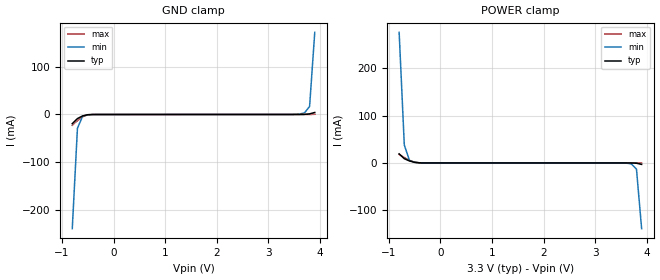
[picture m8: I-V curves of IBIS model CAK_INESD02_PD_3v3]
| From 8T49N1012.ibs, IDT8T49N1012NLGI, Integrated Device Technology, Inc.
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| 3.25758e+00   -2.17677e-02   -5.28452e-01   -1.11757e-02
| 3.33333e+00   -5.02723e-02   -7.41922e-01   -2.21158e-02
| 3.40909e+00   -2.62314e-01   -9.55756e-01   -3.46040e-02
| 3.48485e+00   -5.48303e-01   -1.16986e+00   -4.62037e-02
| 3.56061e+00   -8.34641e-01   -1.38418e+00   -9.03765e-02
| 3.63636e+00   -1.12130e+00   -1.59869e+00   -4.17028e-01
| 3.71212e+00   -1.40825e+00   -1.81339e+00   -7.83888e-01
| 3.78788e+00   -1.69546e+00   -2.02826e+00   -1.15108e+00
| 3.86364e+00   -1.98293e+00   -2.24329e+00   -1.51857e+00
| 3.93939e+00   -2.27062e+00   -2.45848e+00   -1.88632e+00
| 4.01515e+00   -2.55852e+00   -2.67383e+00   -2.25428e+00
| 4.09091e+00   -2.84661e+00   -2.88932e+00   -2.62244e+00
| 4.16667e+00   -3.13486e+00   -3.10494e+00   -2.99075e+00
| 4.24242e+00   -3.42327e+00   -3.32071e+00   -3.35921e+00
| 4.31818e+00   -3.71181e+00   -3.53659e+00   -3.72777e+00
| 4.39394e+00   -4.00047e+00   -3.75260e+00   -4.09645e+00
| 4.46970e+00   -4.28924e+00   -3.96871e+00   -4.46521e+00
| 4.54545e+00   -4.57811e+00   -4.18494e+00   -4.83406e+00
| 4.62121e+00   -4.86706e+00   -4.40126e+00   -5.20297e+00
| 4.69697e+00   -5.15608e+00   -4.61767e+00   -5.57195e+00
| 4.77273e+00   -5.44517e+00   -4.83417e+00   -5.94098e+00
| 4.84848e+00   -5.73432e+00   -5.05076e+00   -6.31005e+00
| 4.92424e+00   -6.02353e+00   -5.26742e+00   -6.67914e+00
| 5.00000e+00   -6.31277e+00   -5.48416e+00   -7.04826e+00
[Model] CAK_INESD02_PD_3v3
Model_type   Input
Polarity   Non-Inverting
Vinl = 0.8V
Vinh = 2.0V
|   typ   min   max
C_comp   2pF   1.5pF   2.5pF
|   typ   min   max
[Voltage range]   3.3V   3.135V   3.465V
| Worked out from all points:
|   GND clamp passes 1 mA (typ) near -0.52 V on its own axis
|   POWER clamp passes 1 mA (typ) near -0.47 V on its own axis
[GND_clamp]
|Voltage   I (typ)   I (min)   I (max)
|Note, modeling breaks down at 250mA and above.  This is well beyond the functional   |
|operating range of the device.  Should this scenario occur, catastrophic failure and   |
|possible damage to the device and/or board is of higher concern than the I-V curve   |
|behavior.  The IBIS checker will flag currents in excess of 10A with warnings.  Lines   |
|with currents in excess of 0.35 A have been commented out.  The points still remain|
|available to the user if the user desires to use them.   |
|-3.30000e+00   -9.17988e+00   -7.26773e+00   -1.13298e+01
|-3.20000e+00   -8.80345e+00   -6.98545e+00   -1.08492e+01
|-3.10000e+00   -8.42702e+00   -6.70323e+00   -1.03687e+01
|-3.00000e+00   -8.05061e+00   -6.42105e+00   -9.88820e+00
|-2.90000e+00   -7.67421e+00   -6.13893e+00   -9.40766e+00
|-2.80000e+00   -7.29783e+00   -5.85686e+00   -8.92712e+00
|-2.70000e+00   -6.92147e+00   -5.57486e+00   -8.44657e+00
|-2.60000e+00   -6.54514e+00   -5.29293e+00   -7.96602e+00
|-2.50000e+00   -6.16885e+00   -5.01107e+00   -7.48547e+00
|-2.40000e+00   -5.79260e+00   -4.72930e+00   -7.00493e+00
|-2.30000e+00   -5.41640e+00   -4.44761e+00   -6.52441e+00
|-2.20000e+00   -5.04025e+00   -4.16601e+00   -6.04391e+00
|-2.10000e+00   -4.66418e+00   -3.88451e+00   -5.56345e+00
|-2.00000e+00   -4.28819e+00   -3.60313e+00   -5.08304e+00
|-1.90000e+00   -3.91230e+00   -3.32186e+00   -4.60270e+00
|-1.80000e+00   -3.53652e+00   -3.04073e+00   -4.12245e+00
|-1.70000e+00   -3.16087e+00   -2.75973e+00   -3.64230e+00
|-1.60000e+00   -2.78537e+00   -2.47887e+00   -3.16225e+00
|-1.50000e+00   -2.41006e+00   -2.19818e+00   -2.68233e+00
|-1.40000e+00   -2.03494e+00   -1.91765e+00   -2.20257e+00
|-1.30000e+00   -1.66006e+00   -1.63729e+00   -1.72300e+00
|-1.20000e+00   -1.28544e+00   -1.35712e+00   -1.24366e+00
|-1.10000e+00   -9.11109e-01   -1.07716e+00   -7.64616e-01
|-1.00000e+00   -5.37100e-01   -7.97430e-01   -2.85915e-01
|-9.00000e-01   -1.63453e-01   -5.18026e-01   -3.47484e-02
-800mV    -19.19mA   -239.1mA   -22.58mA
-700mV    -8.549mA   -28.91mA   -12.7mA
-600mV    -2.981mA   -3.644mA   -4.608mA
-500mV    -492.6uA   -557.5uA   -705.1uA
-400mV    -39.98uA   -64.81uA   -42.86uA
3.4V      67.73uA    64.5uA     78.25uA
3.6V      76.73uA    847.2uA    82.85uA
3.7V      207.4uA    3.364mA    85.29uA
3.8V      1.306mA    16.87mA    99.57uA
3.9V      4.206mA    171.9mA    465.4uA
| 4.00000e+00   9.03254e-03   4.59154e-01   2.65396e-03
| 4.10000e+00   1.91269e-02   7.45979e-01   7.16235e-03
| 4.20000e+00   1.92456e-01   1.03300e+00   1.37928e-02
| 4.30000e+00   5.75454e-01   1.32026e+00   2.02391e-02
| 4.40000e+00   9.58763e-01   1.60777e+00   5.14955e-02
| 4.50000e+00   1.34241e+00   1.89553e+00   4.81824e-01
| 4.60000e+00   1.72638e+00   2.18354e+00   9.72138e-01
| 4.70000e+00   2.11068e+00   2.47179e+00   1.46287e+00
| 4.80000e+00   2.49530e+00   2.76029e+00   1.95401e+00
| 4.90000e+00   2.88022e+00   3.04903e+00   2.44553e+00
| 5.00000e+00   3.26545e+00   3.33802e+00   2.93743e+00
| 5.10000e+00   3.65097e+00   3.62726e+00   3.42970e+00
| 5.20000e+00   4.03679e+00   3.91674e+00   3.92230e+00
| 5.30000e+00   4.42288e+00   4.20647e+00   4.41524e+00
| 5.40000e+00   4.80925e+00   4.49646e+00   4.90850e+00
| 5.50000e+00   5.19591e+00   4.78670e+00   5.40206e+00
| 5.60000e+00   5.58284e+00   5.07721e+00   5.89593e+00
| 5.70000e+00   5.97004e+00   5.36800e+00   6.39009e+00
| 5.80000e+00   6.35753e+00   5.65906e+00   6.88453e+00
| 5.90000e+00   6.74530e+00   5.95041e+00   7.37926e+00
| 6.00000e+00   7.13335e+00   6.24207e+00   7.87427e+00
| 6.10000e+00   7.52170e+00   6.53404e+00   8.36956e+00
| 6.20000e+00   7.91035e+00   6.82634e+00   8.86513e+00
| 6.30000e+00   8.29930e+00   7.11898e+00   9.36099e+00
| 6.40000e+00   8.68858e+00   7.41197e+00   9.85714e+00
| 6.50000e+00   9.07819e+00   7.70534e+00   1.03536e+01
| 6.60000e+00   9.46815e+00   7.99910e+00   1.08503e+01
[Power_clamp]
|Voltage   I (typ)   I (min)   I (max)
|Note, modeling breaks down at 250mA and above.  This is well beyond the functional   |
|operating range of the device.  Should this scenario occur, catastrophic failure and   |
|possible damage to the device and/or board is of higher concern than the I-V curve   |
|behavior.  The IBIS checker will flag currents in excess of 10A with warnings.  Lines   |
|with currents in excess of 0.35 A have been commented out.  The points still remain|
|available to the user if the user desires to use them.   |
|-3.30000e+00   9.46815e+00   7.51754e+00   1.16707e+01
|-3.20000e+00   9.07819e+00   7.22441e+00   1.11734e+01
|-3.10000e+00   8.68858e+00   6.93165e+00   1.06764e+01
|-3.00000e+00   8.29930e+00   6.63923e+00   1.01798e+01
|-2.90000e+00   7.91035e+00   6.34714e+00   9.68345e+00
|-2.80000e+00   7.52170e+00   6.05537e+00   9.18740e+00
|-2.70000e+00   7.13335e+00   5.76391e+00   8.69165e+00
|-2.60000e+00   6.74530e+00   5.47275e+00   8.19617e+00
|-2.50000e+00   6.35753e+00   5.18186e+00   7.70098e+00
|-2.40000e+00   5.97004e+00   4.89125e+00   7.20607e+00
|-2.30000e+00   5.58284e+00   4.60091e+00   6.71144e+00
|-2.20000e+00   5.19591e+00   4.31084e+00   6.21710e+00
|-2.10000e+00   4.80925e+00   4.02101e+00   5.72304e+00
|-2.00000e+00   4.42288e+00   3.73144e+00   5.22928e+00
|-1.90000e+00   4.03679e+00   3.44212e+00   4.73582e+00
|-1.80000e+00   3.65097e+00   3.15304e+00   4.24268e+00
|-1.70000e+00   3.26545e+00   2.86421e+00   3.74985e+00
|-1.60000e+00   2.88022e+00   2.57562e+00   3.25737e+00
|-1.50000e+00   2.49530e+00   2.28728e+00   2.76523e+00
|-1.40000e+00   2.11068e+00   1.99919e+00   2.27345e+00
|-1.30000e+00   1.72638e+00   1.71134e+00   1.78206e+00
|-1.20000e+00   1.34241e+00   1.42374e+00   1.29107e+00
|-1.10000e+00   9.58763e-01   1.13639e+00   8.00480e-01
|-1.00000e+00   5.75454e-01   8.49280e-01   3.10313e-01
|-9.00000e-01   1.92456e-01   5.62397e-01   2.81521e-02
-800mV    19.13mA    275.5mA    18.18mA
-700mV    9.033mA    37.64mA    11.28mA
-600mV    4.206mA    5.523mA    5.325mA
-500mV    1.306mA    1.444mA    1.62mA
-300mV    76.73uA    75.42uA    89.71uA
3.5V      -4.008uA   -29.94uA   -806.4nA
3.7V      -39.97uA   -1.889mA   -5.434uA
3.8V      -492.6uA   -12.86mA   -10.27uA
3.9V      -2.981mA   -138.6mA   -119.5uA
